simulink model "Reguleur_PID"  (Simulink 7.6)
settings: Solver=ode15s  StartTime=0.0  StopTime=20  RelTol=1e-6
InitFcn:
  | clc
StopFcn:
  | close all
  | load Signaux_PID.mat
  | plot(x(1,:),x(2,:),'*',x(1,:),x(3,:),x(1,:),x(4,:))
  | axis([0 20 -0.2 1.2])
  | title('Signaux de consigne, commande et sortie')
  | xlabel('temps')
  | grid
libraries: fl_lib x8, nesl_utility x4, AppliElectrical_lib x1

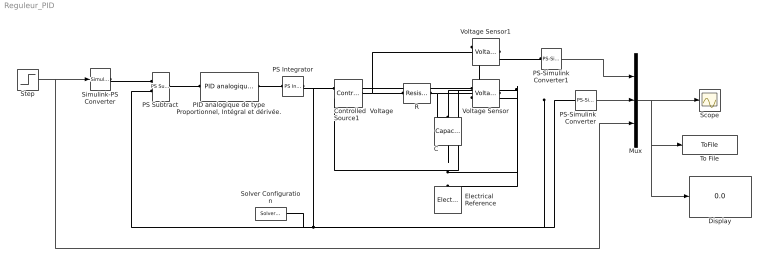
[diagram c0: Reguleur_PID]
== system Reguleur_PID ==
  C : fl_lib/Electrical/Electrical Elements/Capacitor  DialogController=NetworkEngine.DynNeDlgSource  SystemSampleTime=-1  c=1e-6 F  v0=0 V  r=1e-6 Ohm  g=0 1/Ohm  i_Log=off  v_Log=off  vc_Log=off  LocalVarNames=|i|v|vc  LocalVarDescs=|i|v|Internal variable for voltage across capacitor term  LocalVarLogging=[0 0 0]
  Controlled  Voltage Source1 : fl_lib/Electrical/Electrical Sources/Controlled Voltage Source  DialogController=NetworkEngine.DynNeDlgSource  SystemSampleTime=-1  i_Log=off  v_Log=off  LocalVarNames=|i|v  LocalVarDescs=|i|v  LocalVarLogging=[0 0]
  Display : Display
  Electrical Reference : fl_lib/Electrical/Electrical Elements/Electrical Reference  DialogController=NetworkEngine.DynNeDlgSource  SystemSampleTime=-1  i_Log=off  LocalVarNames=|i  LocalVarDescs=|i  LocalVarLogging=0
  Mux : Mux  Inputs=3
  "PID analogique de type Proportionnel, Intégral et dérivée." : AppliElectrical_lib/PID analogique de type Proportionnel, Intégral et dérivée.  DialogController=NetworkEngine.DynNeDlgSource  SystemSampleTime=-1  Kp=0.05  Ki=0.5 1/s  Kd=0.01 s  deriv_Log=off  erreur_Log=off  LocalVarNames=|deriv|erreur  LocalVarDescs=|derr/dt;|err(t);  LocalVarLogging=[0 0]
  PS Integrator : fl_lib/Physical Signals/Linear Operators/PS Integrator  DialogController=NetworkEngine.DynNeDlgSource  SystemSampleTime=-1  x0=0  x_Log=off  LocalVarNames=|x  LocalVarDescs=|x  LocalVarLogging=0
  PS Subtract : fl_lib/Physical Signals/Functions/PS Subtract  DialogController=NetworkEngine.DynNeDlgSource  SystemSampleTime=-1  LocalVarLogging=[]
  PS-Simulink Converter : nesl_utility/PS-Simulink Converter  DialogController=NetworkEngine.DynNeUtilDlgSource  SystemSampleTime=-1  PhysicalDomain=network_engine_domain  LeftPortType=input  RightPortType=output  SubClassName=ps_output  Unit=1  AffineConversion=off
  PS-Simulink Converter1 : nesl_utility/PS-Simulink Converter  DialogController=NetworkEngine.DynNeUtilDlgSource  SystemSampleTime=-1  PhysicalDomain=network_engine_domain  LeftPortType=input  RightPortType=output  SubClassName=ps_output  Unit=1  AffineConversion=off
  R : fl_lib/Electrical/Electrical Elements/Resistor  DialogController=NetworkEngine.DynNeDlgSource  SystemSampleTime=-1  R=1e6 Ohm  i_Log=off  v_Log=off  LocalVarNames=|i|v  LocalVarDescs=|i|v  LocalVarLogging=[0 0]
  Scope : Scope
  Simulink-PS Converter : nesl_utility/Simulink-PS Converter  DialogController=NetworkEngine.DynNeUtilDlgSource  SystemSampleTime=-1  PhysicalDomain=network_engine_domain  LeftPortType=input  RightPortType=output  SubClassName=ps_input  Unit=1  AffineConversion=off  InputFilterTimeConstant=.001  UdotUserProvided=0
  Solver Configuration : nesl_utility/Solver Configuration  DialogController=NetworkEngine.DynNeUtilDlgSource  SystemSampleTime=-1  PhysicalDomain=network_engine_domain  LeftPortType=input  RightPortType=generic  SubClassName=solver  Accelerate=off  Profile=off  ResidualTolerance=1e-9  MaxNonlinIter=3  MaxModeIter=2  DoFixedCost=off  UseLocalSampling=off  DoDC=off  LinearAlgebra=Sparse  LocalSolverSampleTime=.001  LocalSolverChoice=NE_BACKWARD_EULER_ADVANCER  UseLocalSolver=off
  Step : Step  Time=5  SampleTime=0
  To File : ToFile  Filename=Signaux_PID  MatrixName=x
  Voltage Sensor : fl_lib/Electrical/Electrical Sensors/Voltage Sensor  DialogController=NetworkEngine.DynNeDlgSource  SystemSampleTime=-1  i1_Log=off  v1_Log=off  LocalVarNames=|i1|v1  LocalVarDescs=|i1|v1  LocalVarLogging=[0 0]
  Voltage Sensor1 : fl_lib/Electrical/Electrical Sensors/Voltage Sensor  DialogController=NetworkEngine.DynNeDlgSource  SystemSampleTime=-1  i1_Log=off  v1_Log=off  LocalVarNames=|i1|v1  LocalVarDescs=|i1|v1  LocalVarLogging=[0 0]
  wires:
  Step/1 -> Simulink-PS Converter/1, Mux/3
  Mux/1 -> Scope/1, To File/1, Display/1
  PS-Simulink Converter/1 -> Mux/2
  PS-Simulink Converter1/1 -> Mux/1
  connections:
  PS Subtract/RConn1 -- "PID analogique de type Proportionnel, Intégral et dérivée."/LConn1
  Controlled  Voltage Source1/RConn2 -- Electrical Reference/LConn1 -- C/RConn1 -- Voltage Sensor/RConn2 -- Voltage Sensor1/RConn2
  R/RConn1 -- C/LConn1 -- Voltage Sensor/LConn1
  Simulink-PS Converter/RConn1 -- PS Subtract/LConn1
  PS-Simulink Converter/LConn1 -- Voltage Sensor/RConn1 -- PS Subtract/LConn2 -- Solver Configuration/RConn1
  Controlled  Voltage Source1/LConn1 -- R/LConn1 -- Voltage Sensor1/LConn1
  PS Integrator/RConn1 -- Controlled  Voltage Source1/RConn1
  "PID analogique de type Proportionnel, Intégral et dérivée."/RConn1 -- PS Integrator/LConn1
  Voltage Sensor1/RConn1 -- PS-Simulink Converter1/LConn1
